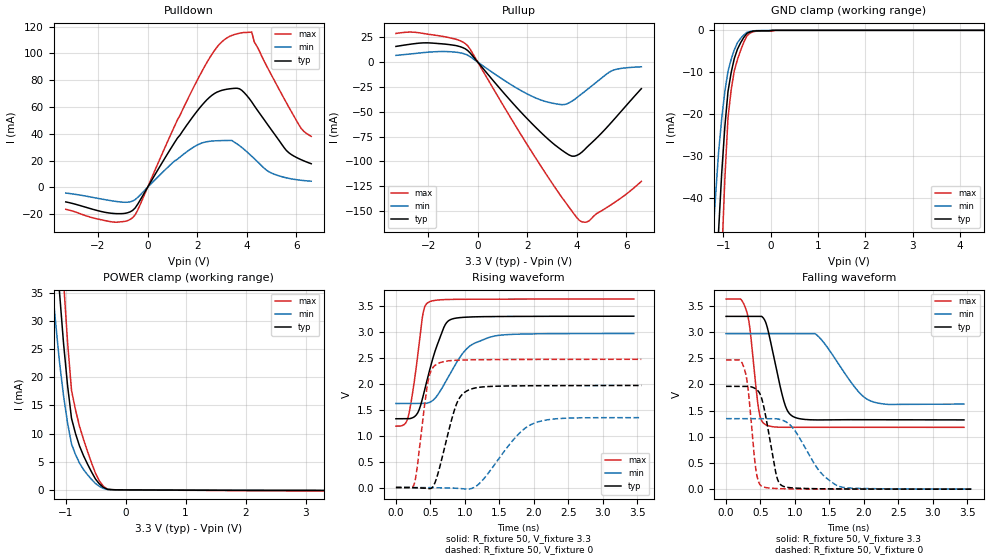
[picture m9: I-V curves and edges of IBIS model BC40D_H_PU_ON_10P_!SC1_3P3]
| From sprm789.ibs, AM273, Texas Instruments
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|   Model Cell BC40D_H_PU_ON_10P_!SC1_3P3
|BC40D_H_PU_ON_10P_!SC1_3P3
[Model]   BC40D_H_PU_ON_10P_!SC1_3P3
Model_type   I/O
Polarity   Non-Inverting
Enable   Active-Low
Vinl =  0.8V
Vinh =  2V
Cref =  15pF
Rref =  100.0000M
Vref =  0V
Vmeas =  1.65
C_comp   2.157014p   1.997104p   2.250886p
|[Input load] weak_pu_on
|[Output drive] fast
|[supplytol] 10
|[temp] ind
[Model Spec]
Vinl   0.8V   0.8V   0.8V
Vinh   2V   2V   2V
[Temperature Range]   25   125   -40
[Voltage Range]   3.3   2.97   3.63
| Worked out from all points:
|   slope of the pulldown table from 0 to 0.495 V, typ, clamps not added: 31.8 ohm
|   slope of the pullup table from 0 to 0.495 V, typ, clamps not added: 33.3 ohm
|   GND clamp passes 1 mA (typ) near -0.52 V on its own axis
|   POWER clamp passes 1 mA (typ) near -0.43 V on its own axis
|   rising waveform, R_fixture 50, V_fixture 3.3: 20-80 % time 258ps typ, 390ps min, 146ps max; typ from 1.32 V to 3.3 V
|   rising waveform, R_fixture 50, V_fixture 0: 20-80 % time 233ps typ, 479ps min, 138ps max; typ from 0 V to 1.97 V
|   falling waveform, R_fixture 50, V_fixture 3.3: 20-80 % time 199ps typ, 427ps min, 119ps max; typ from 3.3 V to 1.32 V
|   falling waveform, R_fixture 50, V_fixture 0: 20-80 % time 162ps typ, 386ps min, 107ps max; typ from 1.96 V to 0.003 V
| Nom Voltages:
|   VDD=1.1001, VDDS=3.3, VDDS18=1.8, ESD_BIASFET=0, VSS=0, VSSS=0
| Min Voltages:
|   VDD=0.99, VDDS=2.97, VDDS18=1.62, ESD_BIASFET=0, VSS=0, VSSS=0
| Max Voltages:
|   VDD=1.21, VDDS=3.63, VDDS18=1.98, ESD_BIASFET=0, VSS=0, VSSS=0
[POWER_clamp]
|   voltage   I(typ)   I(min)   I(max)
-3.3V     446.9mA    419.5mA    603.9mA
-1.233V   56.55mA    37.52mA    80.26mA
-1.167V   45.63mA    29.9mA     65.05mA
-1.1V     35.1mA     22.66mA    50.24mA
-1.033V   26.08mA    16.76mA    37.18mA
-966.7mV  18.62mA    11.92mA    26.33mA
-900mV    12.7mA     8.149mA    17.69mA
-833.3mV  10mA       6.265mA    14.21mA
-766.7mV  7.795mA    4.753mA    11.3mA
-566.7mV  3.199mA    1.871mA    4.823mA
-366.7mV  433.5uA    268.4uA    618.3uA
3.3V      -100.3uA   -83.23uA   -188.3uA
[Pulldown]
|   voltage   I(typ)   I(min)   I(max)
-3.3V     -10.92mA   -4.307mA   -16.45mA
-1.4V     -19.52mA   -10.22mA   -25.94mA
-600mV    -17.22mA   -10.25mA   -22.66mA
1.1V      33.8mA     19.88mA    46.22mA
2.1V      59.3mA     32.44mA    83.48mA
2.9V      71.86mA    34.84mA    107mA
3.5V      73.95mA    33.66mA    114.2mA
4.2V      63.8mA     23.19mA    116mA
4.9V      45.33mA    11.53mA    87.2mA
5.6V      27.47mA    7.046mA    63.1mA
6.2V      20.56mA    5.221mA    43.87mA
6.6V      17.6mA     4.555mA    38.05mA
[Pullup]
|   voltage   I(typ)   I(min)   I(max)
-3.3V     15.77mA    6.741mA    28.8mA
-1.9V     19.23mA    10.15mA    27.67mA
-900mV    16.69mA    10.02mA    23.17mA
-400mV    11.53mA    6.853mA    16.25mA
1.3V      -38.16mA   -22.04mA   -54.88mA
2.3V      -64.7mA    -35.66mA   -95.04mA
3.4V      -88.76mA   -42.82mA   -136.4mA
3.8V      -94.64mA   -39.36mA   -150mA
4.1V      -92.53mA   -33.79mA   -159.3mA
4.4V      -85.77mA   -27.94mA   -161mA
5.4V      -60.46mA   -8.849mA   -143.2mA
6.6V      -26.71mA   -4.741mA   -120mA
[GND_clamp]
|   voltage   I(typ)   I(min)   I(max)
-3.3V     -787.2mA   -607.8mA   -1.235A
-1.233V   -85.67mA   -52.14mA   -138.8mA
-1.167V   -66.48mA   -40.37mA   -107.8mA
-1.1V     -48.26mA   -29.37mA   -78.02mA
-1.033V   -34.3mA    -21.2mA    -54.63mA
-966.7mV  -23.1mA    -14.67mA   -35.61mA
-900mV    -14.66mA   -9.802mA   -20.96mA
-833.3mV  -10.12mA   -6.954mA   -14.3mA
-700mV    -4.501mA   -2.964mA   -6.982mA
-500mV    -717.7uA   -486.4uA   -1.28mA
100mV     0A         0A         0A
6.6V      0A         0A         0A
[Ramp]
| variable   typ   min   max
dV/dt_f  1.1950017/0.20080866n 0.83559507/0.44366737n  1.4746419/0.11970936n
dV/dt_r  1.1920125/0.23572139n 0.82832286/0.49069736n  1.4896526/0.13868874n
R_load = 50
[Rising Waveform]
R_fixture = 50
V_fixture = 3.3
V_fixture_min = 2.97
V_fixture_max = 3.63
|   time   V(typ)   V(min)   V(max)
0s        1.324V     1.618V     1.183V
178.4ps   1.324V     1.618V     1.364V
304.9ps   1.415V     1.618V     2.418V
390.3ps   1.738V     1.618V     3.33V
473.9ps   2.182V     1.633V     3.569V
694.3ps   3.08V      1.973V     3.619V
826.1ps   3.25V      2.286V     3.624V
1.071ns   3.284V     2.723V     3.627V
1.437ns   3.293V     2.919V     3.628V
3.453ns   3.299V     2.966V     3.63V
[Rising Waveform]
R_fixture = 50
V_fixture = 0
V_fixture_min = 0
V_fixture_max = 0
|   time   V(typ)   V(min)   V(max)
0s        0V         0V         2.623mV
263.8ps   -3.484mV   0V         59.42mV
303.3ps   -5.333mV   0V         335.2mV
467.3ps   -18.71mV   0V         2.052V
607.9ps   258mV      -4.352mV   2.387V
870.5ps   1.577V     -13.71mV   2.451V
1.053ns   1.876V     -30.55mV   2.458V
1.23ns    1.934V     101.3mV    2.462V
1.988ns   1.96V      1.229V     2.467V
3.563ns   1.965V     1.346V     2.469V
[Falling Waveform]
R_fixture = 50
V_fixture = 3.3
V_fixture_min = 2.97
V_fixture_max = 3.63
|   time   V(typ)   V(min)   V(max)
0s        3.299V     2.969V     3.629V
297.2ps   3.299V     2.969V     3.4V
345.6ps   3.299V     2.969V     3.075V
475.2ps   3.299V     2.969V     1.512V
572.9ps   3.193V     2.969V     1.234V
839.6ps   1.679V     2.969V     1.183V
979.5ps   1.383V     2.969V     1.183V
1.329ns   1.323V     2.931V     1.183V
2.099ns   1.326V     1.685V     1.182V
3.453ns   1.324V     1.626V     1.182V
[Falling Waveform]
R_fixture = 50
V_fixture = 0
V_fixture_min = 0
V_fixture_max = 0
|   time   V(typ)   V(min)   V(max)
0s        1.964V     1.348V     2.469V
269.9ps   1.964V     1.348V     2.28V
325ps     1.963V     1.348V     1.854V
432ps     1.915V     1.348V     382.7mV
521.9ps   1.713V     1.348V     56.24mV
730ps     270.2mV    1.345V     14.61mV
830ps     57.47mV    1.312V     9.704mV
1.375ns   9.578mV    317.2mV    3.884mV
1.632ns   7.347mV    60.06mV    3.359mV
3.563ns   2.505mV    4.298mV    3.076mV
